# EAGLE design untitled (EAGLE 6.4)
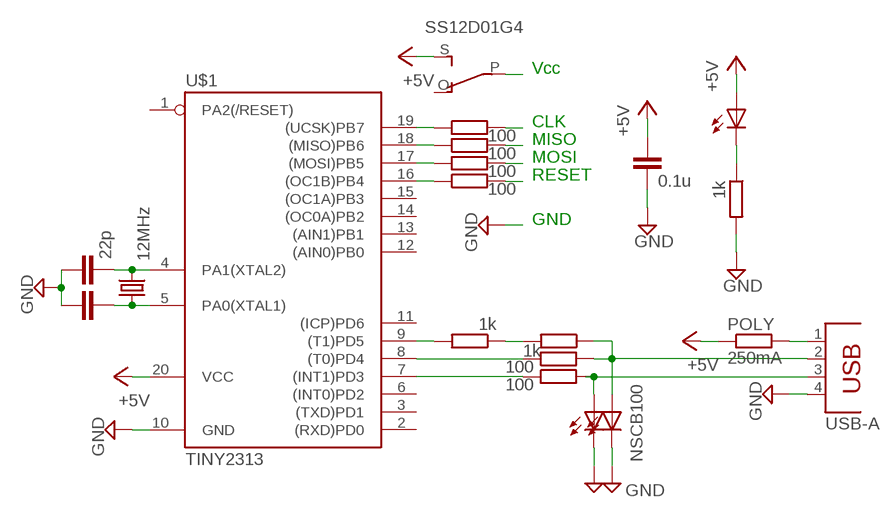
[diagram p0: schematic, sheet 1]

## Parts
C1  22p  C-EUC2012  [C2012]
C2  22p  C-EUC2012  [C2012]
C3  0.1u  C-EUC2012  [C2012]
LED1  NSCB100  LED3020  [CHIPLED_3020]
LED2  NSCB100  LED3020  [CHIPLED_3020]
LED3  LED3MM  [LED3MM]
POLY  250mA  R-EU_0204/5  [0204/5]
Q2  12MHz  CRYSTALHC49S  [HC49/S]
R1  100  R-EU_R2012  [R2012]
R2  100  R-EU_R2012  [R2012]
R3  1k  R-EU_R2012  [R2012]
R4  1k  R-EU_R2012  [R2012]
R5  1k  R-EU_R2012  [R2012]
R7  100  R-EU_R2012  [R2012]
R8  100  R-EU_R2012  [R2012]
R9  100  R-EU_R2012  [R2012]
R10  100  R-EU_R2012  [R2012]
U$1  TINY2313  [DIL20$]
U$2  USB-A  [USB_A]
U$4  SS12D01G4  [SS12D01G4]

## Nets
+5V: C3.1 LED3.A POLY.1 U$1.20(VCC) U$4.S
GND: C1.1 C2.1 C3.2 LED1.C LED2.C R4.2 U$1.10(GND) U$2.4
N$1: R1.1 U$1.8((T0)PD4)
N$2: R2.1 U$1.7((INT1)PD3)
N$3: LED1.A R1.2 R5.1 U$2.2
N$4: R7.1 U$1.19((UCSK)PB7)
N$5: U$4.P
N$6: C2.2 Q2.2 U$1.4(PA1(XTAL2))
N$7: C1.2 Q2.1 U$1.5(PA0(XTAL1))
N$8: POLY.2 U$2.1
N$10: LED2.A R2.2 U$2.3
N$11: R3.1 R5.2
N$12: R3.2 U$1.9((T1)PD5)
N$16: LED3.K(C) R4.1
N$19: R7.2
N$21: R8.1 U$1.18((MISO)PB6)
N$22: R9.1 U$1.17((MOSI)PB5)
N$23: R10.1 U$1.16((OC1B)PB4)
N$24: R8.2
N$25: R9.2
N$26: R10.2
Unconnected: U$1.1(PA2(/RESET)) U$1.2((RXD)PD0) U$1.3((TXD)PD1) U$1.6((INT0)PD2) U$1.11((ICP)PD6) U$1.12((AIN0)PB0) U$1.13((AIN1)PB1) U$1.14((OC0A)PB2) U$1.15((OC1A)PB3) U$4.O

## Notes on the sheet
- Vcc
- CLK
- MISO
- MOSI
- RESET
- GND

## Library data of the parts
C1-C3 = rcl:C-EU: CAPACITOR, European symbol
LED1-LED3 = led:LED: LED
POLY = resistor:R-EU_: RESISTOR, European symbol
Q2 = crystal:CRYSTAL: CRYSTAL
R1-R5 R7-R10 = rcl:R-EU_: RESISTOR, European symbol
U$1 = avr-7:TINY2313*: Atmel Tiny2313 2K Flash, 128 bytes EEPROM, 128 bytes RAM
U$2 = _yskcon's:USB-A
U$4 = _yskcon's:SS12D01G4

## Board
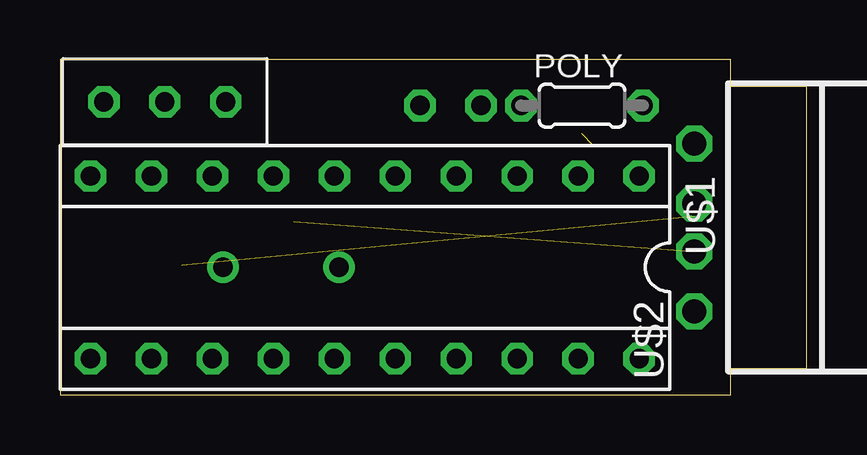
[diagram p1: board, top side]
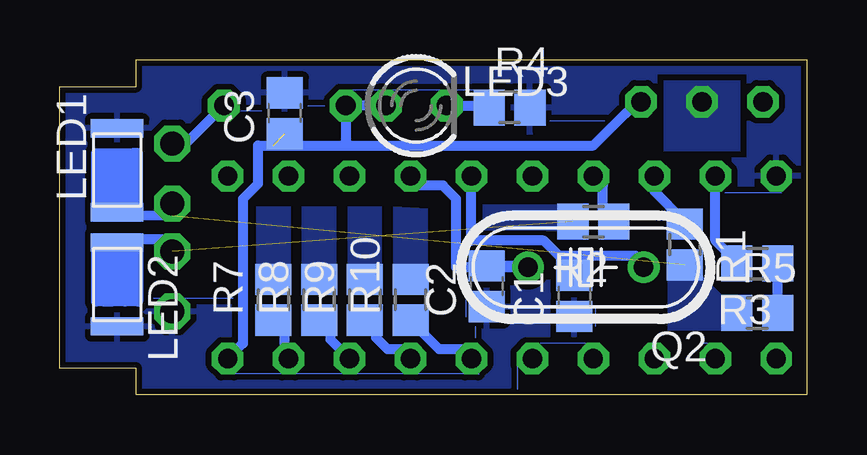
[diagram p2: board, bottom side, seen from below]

Size 31.11 x 13.97 mm. Coordinates in mm from the lower left corner, seen from the top.
Outline: 0,0 27.94,0 27.94,1.11 31.11,1.11 31.11,12.86 27.94,12.86 27.94,13.97 0,13.97 0,0
Copper layers (1*16): Top 0.035mm / dielectric 1.5mm / Bottom 0.035mm
Design rules "default *": minimum track width 10mil, minimum drill 24mil, track to track 8mil, track to pad 8mil, pad to pad 8mil, via to via 8mil, smd to smd 8mil, copper to edge 10mil, drill to drill 8mil, minimum pad ring 10mil, minimum via ring 8mil, stop-mask expansion 4mil, vias tented up to drill 0mil, thermal gap 10mil

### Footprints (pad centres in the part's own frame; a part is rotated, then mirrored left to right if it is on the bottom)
C2012 = smd 1.3 x 1.5: 1 -0.85,0; 2 0.85,0
CHIPLED_3020 = smd 2.184 x 0.762: A 0,-1.75; C 0,1.75
LED3MM = drill 0.813 octagon: A -1.27,0; K 1.27,0
0204/5 = drill 0.813 octagon: 1 -2.54,0; 2 2.54,0
HC49/S = drill 0.813: 1 -2.413,0; 2 2.413,0
R2012 = smd 1.3 x 1.5: 1 -0.85,0; 2 0.85,0
DIL20$ = drill 0.8 octagon: 1 -11.43,-3.81; 2 -8.89,-3.81; 3 -6.35,-3.81; 4 -3.81,-3.81; 5 -1.27,-3.81; 6 1.27,-3.81; 7 3.81,-3.81; 8 6.35,-3.81; 9 8.89,-3.81; 10 11.43,-3.81; 11 11.43,3.81; 12 8.89,3.81; 13 6.35,3.81; 14 3.81,3.81; 15 1.27,3.81; 16 -1.27,3.81; 17 -3.81,3.81; 18 -6.35,3.81; 19 -8.89,3.81; 20 -11.43,3.81
USB_A = drill 1 octagon: 1 3.5,0; 2 1,0; 3 -1,0; 4 -3.5,0
SS12D01G4 = drill 0.8 octagon: O -2.54,0; P 0,0; S 2.54,0

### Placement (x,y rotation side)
C1  9.68,4.13 90 bottom
C2  13.34,4.52 90 bottom
C3  21.75,11.75 90 bottom
LED1  28.73,9.37 0 bottom
LED2  28.73,4.6 180 bottom
LED3  16.27,12.06 0 bottom
POLY  21.75,12.07 0 top
Q2  9.21,5.32 180 bottom
R1  5.08,6.27 270 bottom
R2  8.89,7.22 180 bottom
R3  2.06,5.48 180 bottom
R4  12.38,11.99 0 bottom
R5  2.06,3.41 0 bottom
R7  22.23,3.97 90 bottom
R8  20.32,3.97 90 bottom
R9  18.41,3.97 90 bottom
R10  16.51,3.97 90 bottom
U$1  12.7,5.32 180 top
U$2  26.43,6.99 90 top
U$4  4.37,12.22 0 top

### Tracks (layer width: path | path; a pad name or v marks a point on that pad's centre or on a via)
+5V  (1 unrouted)
  Bottom 0.406: U$1.20 23.5,2.14 23.5,8.18 22.86,8.81 22.86,10.4 22.23,10.4 19.05,10.4 | 19.05,10.4 8.89,10.4 7.54,11.75 U$4.S | LED3.A 18.81,12.06 POLY.1 19.21,10.56 19.05,10.4
GND
  Bottom 0.406: LED2.C 29.52,2.85
  pour Bottom (isolate 0.254, rank 3): -1.27,-3.57 -4.21,18.73 35.8,16.43 35.56,-3.57
N$1
  Bottom 0.406: R1.1 5.14,7.28 6.35,8.49 U$1.8
N$2
  Bottom 0.406: R2.1 8.44,7.64 8.49,7.7 8.49,8.73 U$1.7
N$3  (1 unrouted)
  Bottom 0.406: 2.7,3.36 R5.1 | U$2.2 26.43,7.46 29.5,7.49 29.57,7.57 29.29,7.86 28.26,7.62 | 28.26,7.62 LED1.A | 28.26,7.62 27.86,7.62 27.86,10.08 28.1,10.08 | 29.61,7.86 29.61,10.08 28.1,10.08 | 28.1,10.08 28.1,8.02 29.29,8.02 29.29,9.84 28.34,9.84 28.34,8.26 29.21,8.26 29.21,9.6 28.57,9.6 28.57,8.49 28.97,8.49 28.97,9.29 28.73,9.29
  pour Bottom (no thermals): 4.37,5 5.79,4.84 5.79,2.7 3.49,2.7 3.49,4.13
N$4
  Bottom 0.406: U$1.19 21.75,1.67 21.75,2.64 R7.1
N$5
  pour Bottom (no thermals): 5.95,13.1 5.95,10.16 2.78,10.16 2.78,13.1
N$6
  Bottom 0.406: C2.2 11.54,5.37 Q2.2 14.61,5.32 14.61,8.18 15.16,8.73 16.27,8.73 U$1.4
N$7
  Bottom 0: C1.2 9.68,5.79
  Bottom 0.406: Q2.1 6.79,5.45 7.14,5.79 9.68,5.79 10.32,5.79 10.95,6.43 13.97,6.43 U$1.5
N$8
  Bottom 0.406: POLY.2 25.88,10.48 U$2.1
N$9
  Bottom 0: 12.06,1.27 12.06,0.24
N$10  (1 unrouted)
  Bottom 0.406: 27.91,6.35 27.86,6.35 27.86,3.89 28.42,3.89 | 27.91,6.35 LED2.A | 28.42,3.89 28.97,3.89 | 29.29,3.89 29.61,3.89 29.61,6.03 29.37,6.03 29.29,6.11 29.29,3.89 | 29.29,3.89 28.97,3.89 | 28.97,3.89 28.97,6.03 29.05,6.11 28.73,6.11 28.73,3.97 28.5,3.97 28.42,3.89 | 28.42,3.89 28.42,6.11 28.18,6.11 28.18,4.05 | 27.91,6.35 27.91,6.4 27.94,6.43 27.94,6.51 26.51,6.51 U$2.3
  pour Bottom (no thermals): 13.49,6.83 13.49,7.94 10.16,7.94 10.16,6.91 10.4,6.83
N$11
  Bottom 0.406: R5.2 R3.1
N$12
  Bottom 0.406: R3.2 2.91,5.53 3.81,6.43 U$1.9
N$13
  Bottom 0: 13.81,0.87 13.65,0.87
N$14
  Bottom 0: 27.23,4.05 23.89,4.05
N$16
  Bottom 0.406: LED3.K 13.31,12.06 R4.1
N$17
  Bottom 0: 4.13,2.14 4.45,2.14
N$18
  Bottom 0: 14.21,3.97 14.21,3.25
N$19
  Bottom 0.406: 21.8,4.68 R7.2
  pour Bottom (no thermals): 21.51,5.32 21.51,7.86 22.94,7.86 22.94,5.32
N$20
  Bottom 0: 14.29,0.87 23.81,0.87
N$21
  Bottom 0.406: U$1.18 19.84,2.3 19.84,2.64 R8.1
N$22
  Bottom 0.406: U$1.17 16.51,1.91 17.46,1.91 17.94,2.38 17.94,2.64 R9.1
N$23
  Bottom 0.406: U$1.16 13.97,1.91 15.32,1.91 16.03,2.62 16.03,2.64 R10.1
N$24
  pour Bottom (no thermals): 19.61,5.32 19.61,7.86 21.03,7.86 21.03,5.32
N$25
  pour Bottom (no thermals): 17.7,5.4 17.7,7.86 19.13,7.86 19.13,5.4
N$26
  pour Bottom (no thermals): 15.8,5.32 15.8,7.78 17.22,7.86 17.22,5.4
N$27
  Bottom 0: 13.89,12.7 19.05,12.7
N$28
  Bottom 0: 22.7,11.83 23.57,11.83
N$29
  Bottom 0: 20.8,12.06 20.08,12.06
N$30
  Bottom 0: 1.03,8.41 3.41,8.41
N$31
  Bottom 0: 8.81,3.65 8.81,2.86
N$32
  Bottom 0: 10.72,11.43 8.41,11.43
N$33
  Bottom 0: 13.81,2.86 13.81,2.38
N$34
  Bottom 0: 9.21,2.14 11.11,2.14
